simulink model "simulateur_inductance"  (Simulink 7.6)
settings: Solver=ode15s  StartTime=0.0  StopTime=200  RelTol=1e-3
InitFcn:
  | clear all, clc
  | R1=1e3;
  | R2=R1;
  | R=R1;
  | C=10e-3;
StopFcn:
  | close all, clc
  | load simul_inductance.mat
  | plot(x(1,:),x(2,:),x(1,:),x(3,:))
  | title('Tension inductance simulée et circuit équivalent')
  | axis([0 200 -0.05 0.4])
  | xlabel('temps')
  | grid
  | delete *.mat
libraries: fl_lib x14, nesl_utility x4, elec_lib x1

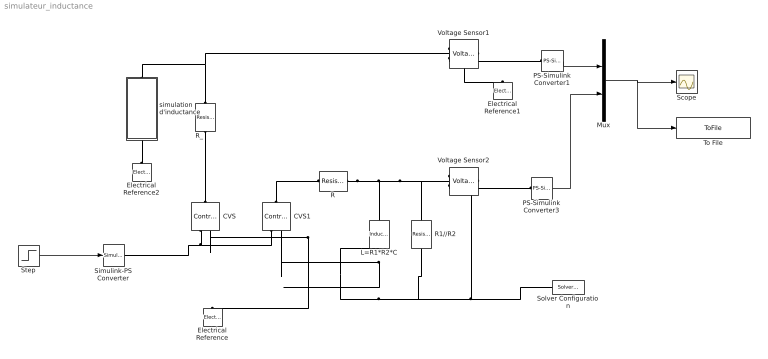
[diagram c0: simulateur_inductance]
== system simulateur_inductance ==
  CVS : fl_lib/Electrical/Electrical Sources/Controlled Voltage Source  DialogController=NetworkEngine.DynNeDlgSource  SystemSampleTime=-1  i_Log=off  v_Log=off  LocalVarNames=|i|v  LocalVarDescs=|i|v  LocalVarLogging=[0 0]
  CVS1 : fl_lib/Electrical/Electrical Sources/Controlled Voltage Source  DialogController=NetworkEngine.DynNeDlgSource  SystemSampleTime=-1  i_Log=off  v_Log=off  LocalVarNames=|i|v  LocalVarDescs=|i|v  LocalVarLogging=[0 0]
  Electrical Reference : fl_lib/Electrical/Electrical Elements/Electrical Reference  DialogController=NetworkEngine.DynNeDlgSource  SystemSampleTime=-1  i_Log=off  LocalVarNames=|i  LocalVarDescs=|i  LocalVarLogging=[]
  Electrical Reference1 : fl_lib/Electrical/Electrical Elements/Electrical Reference  DialogController=NetworkEngine.DynNeDlgSource  SystemSampleTime=-1  i_Log=off  LocalVarNames=|i  LocalVarDescs=|i  LocalVarLogging=[]
  Electrical Reference2 : fl_lib/Electrical/Electrical Elements/Electrical Reference  DialogController=NetworkEngine.DynNeDlgSource  SystemSampleTime=-1  i_Log=off  LocalVarNames=|i  LocalVarDescs=|i  LocalVarLogging=[]
  L=R1*R2*C : fl_lib/Electrical/Electrical Elements/Inductor  DialogController=NetworkEngine.DynNeDlgSource  SystemSampleTime=-1  l=R1*R2*C H  i0=0 A  r=0 Ohm  g=1e-22 1/Ohm  i_Log=off  v_Log=off  i_L_Log=off  LocalVarNames=|i|v|i_L  LocalVarDescs=|i|v|Internal variable for current through inductor term  LocalVarLogging=[0 0 0]
  Mux : Mux  Inputs=2
  PS-Simulink Converter1 : nesl_utility/PS-Simulink Converter  DialogController=NetworkEngine.DynNeUtilDlgSource  SystemSampleTime=-1  PhysicalDomain=network_engine_domain  LeftPortType=input  RightPortType=output  SubClassName=ps_output  Unit=1  AffineConversion=off
  PS-Simulink Converter3 : nesl_utility/PS-Simulink Converter  DialogController=NetworkEngine.DynNeUtilDlgSource  SystemSampleTime=-1  PhysicalDomain=network_engine_domain  LeftPortType=input  RightPortType=output  SubClassName=ps_output  Unit=1  AffineConversion=off
  R : fl_lib/Electrical/Electrical Elements/Resistor  DialogController=NetworkEngine.DynNeDlgSource  SystemSampleTime=-1  R=R Ohm  i_Log=off  v_Log=off  LocalVarNames=|i|v  LocalVarDescs=|i|v  LocalVarLogging=[0 0]
  R1//R2 : fl_lib/Electrical/Electrical Elements/Resistor  DialogController=NetworkEngine.DynNeDlgSource  SystemSampleTime=-1  R=R1*R2/(R1+R2) Ohm  i_Log=off  v_Log=off  LocalVarNames=|i|v  LocalVarDescs=|i|v  LocalVarLogging=[0 0]
  R_ : fl_lib/Electrical/Electrical Elements/Resistor  DialogController=NetworkEngine.DynNeDlgSource  SystemSampleTime=-1  R=R Ohm  i_Log=off  v_Log=off  LocalVarNames=|i|v  LocalVarDescs=|i|v  LocalVarLogging=[0 0]
  Scope : Scope
  Simulink-PS Converter : nesl_utility/Simulink-PS Converter  DialogController=NetworkEngine.DynNeUtilDlgSource  SystemSampleTime=-1  PhysicalDomain=network_engine_domain  LeftPortType=input  RightPortType=output  SubClassName=ps_input  Unit=1  AffineConversion=off  InputFilterTimeConstant=.001  UdotUserProvided=0
  Solver Configuration : nesl_utility/Solver Configuration  DialogController=NetworkEngine.DynNeUtilDlgSource  SystemSampleTime=-1  PhysicalDomain=network_engine_domain  LeftPortType=input  RightPortType=generic  SubClassName=solver  Accelerate=off  Profile=off  ResidualTolerance=1e-9  MaxNonlinIter=12  MaxModeIter=2  DoFixedCost=off  UseLocalSampling=off  DoDC=off  LinearAlgebra=Sparse  LocalSolverSampleTime=.001  LocalSolverChoice=NE_BACKWARD_EULER_ADVANCER  UseLocalSolver=off
  Step : Step  Time=10  SampleTime=0
  To File : ToFile  Filename=simul_inductance  MatrixName=x
  Voltage Sensor1 : fl_lib/Electrical/Electrical Sensors/Voltage Sensor  DialogController=NetworkEngine.DynNeDlgSource  SystemSampleTime=-1  i1_Log=off  v1_Log=off  LocalVarNames=|i1|v1  LocalVarDescs=|i1|v1  LocalVarLogging=[0 0]
  Voltage Sensor2 : fl_lib/Electrical/Electrical Sensors/Voltage Sensor  DialogController=NetworkEngine.DynNeDlgSource  SystemSampleTime=-1  i1_Log=off  v1_Log=off  LocalVarNames=|i1|v1  LocalVarDescs=|i1|v1  LocalVarLogging=[0 0]
  simulation  d'inductance : Subsystem
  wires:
  PS-Simulink Converter1/1 -> Mux/1
  Step/1 -> Simulink-PS Converter/1
  PS-Simulink Converter3/1 -> Mux/2
  Mux/1 -> Scope/1, To File/1
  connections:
  CVS1/RConn1 -- Simulink-PS Converter/RConn1 -- CVS/RConn1
  Voltage Sensor2/RConn2 -- R1//R2/LConn1 -- L=R1*R2*C/LConn1 -- CVS1/RConn2 -- Electrical Reference/LConn1 -- CVS/RConn2 -- Solver Configuration/RConn1
  Voltage Sensor1/RConn1 -- PS-Simulink Converter1/LConn1
  Voltage Sensor1/RConn2 -- Electrical Reference1/LConn1
  R_/RConn1 -- Voltage Sensor1/LConn1 -- simulation  d'inductance/LConn1
  R/RConn1 -- L=R1*R2*C/RConn1 -- R1//R2/RConn1 -- Voltage Sensor2/LConn1
  Voltage Sensor2/RConn1 -- PS-Simulink Converter3/LConn1
  R_/LConn1 -- CVS/LConn1
  CVS1/LConn1 -- R/LConn1
  simulation  d'inductance/RConn1 -- Electrical Reference2/LConn1

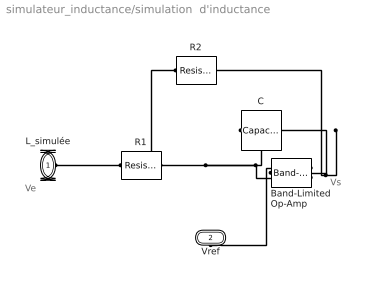
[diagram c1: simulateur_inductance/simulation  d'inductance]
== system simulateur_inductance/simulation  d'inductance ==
  note: Ve
  note: Vs
  Band-Limited Op-Amp : elec_lib/Integrated Circuits/Band-Limited Op-Amp  DialogController=NetworkEngine.DynNeDlgSource  SystemSampleTime=-1  A=1000  Rin=1e+6 Ohm  Rout=100 Ohm  Vmin=-15 V  Vmax=15 V  Vdotmax=1000 V/s  f=1e+5 Hz  V0=0 V  LocalVarLogging=[]
  C : fl_lib/Electrical/Electrical Elements/Capacitor  DialogController=NetworkEngine.DynNeDlgSource  SystemSampleTime=-1  c=C F  v0=0 V  r=1e-22 Ohm  g=0 1/Ohm  i_Log=off  v_Log=off  vc_Log=off  LocalVarNames=|i|v|vc  LocalVarDescs=|i|v|Internal variable for voltage across capacitor term  LocalVarLogging=[0 0 0]
  R1 : fl_lib/Electrical/Electrical Elements/Resistor  DialogController=NetworkEngine.DynNeDlgSource  SystemSampleTime=-1  R=R1 Ohm  i_Log=off  v_Log=off  LocalVarNames=|i|v  LocalVarDescs=|i|v  LocalVarLogging=[0 0]
  R2 : fl_lib/Electrical/Electrical Elements/Resistor  DialogController=NetworkEngine.DynNeDlgSource  SystemSampleTime=-1  R=R2 Ohm  i_Log=off  v_Log=off  LocalVarNames=|i|v  LocalVarDescs=|i|v  LocalVarLogging=[0 0]
  L_simulée : PMIOPort  Port=1  Side=Left
  Vref : PMIOPort  Port=2  Side=Right
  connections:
  Band-Limited Op-Amp/LConn1 -- Vref/RConn1
  R1/RConn1 -- L_simulée/RConn1 -- R2/LConn1
  Band-Limited Op-Amp/RConn1 -- R2/RConn1 -- C/LConn1
  Band-Limited Op-Amp/LConn2 -- C/RConn1 -- R1/LConn1
